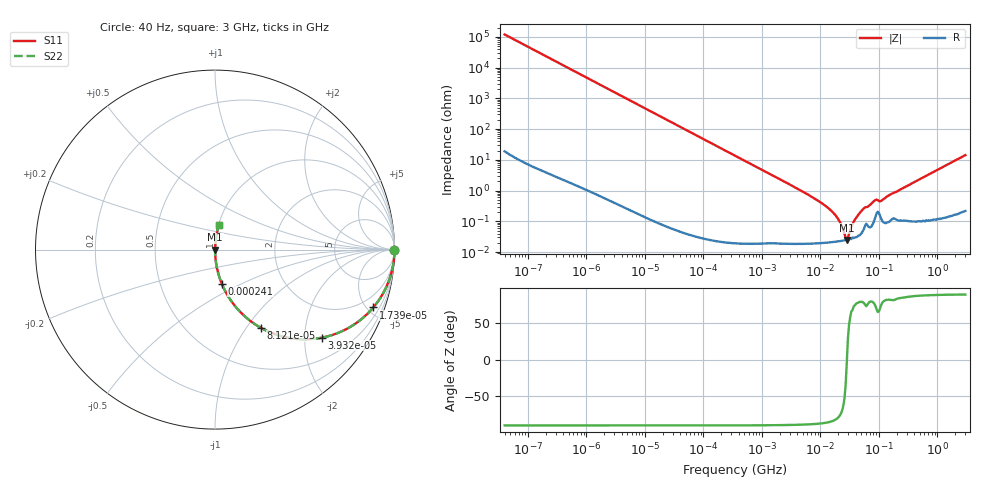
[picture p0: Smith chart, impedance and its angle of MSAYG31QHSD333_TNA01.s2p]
! MSAYG31QHSD333_TNA01  S-PARAMETER MODEL  ( General Type )
! Model Generated by TAIYO YUDEN Corporation (http://www.ty-top.com)
! Version 2.0
! TAIYO YUDEN Control No. 031016
! Copyright(c) 2003 TAIYO YUDEN CO.,LTD. All Rights Reserved.
! Product Description (link to TY-COMPAS)
! https://ds.yuden.co.jp/TYCOMPAS/or/detail?pn=MSAYG31QHSD333KTNA01&u=M
! Products Name : Multilayer Ceramic Capacitors
! Characteristics :
!  Capacitance : 0.033 uF , Rated Voltage : 35V
!  Case Size : 3.2 x 1.6 / 0.126 x 0.063 [mm/inch] , Thickness : 1.15 / 0.045 [mm/inch]
!  (Conditions: Temperature = 25 degC , DC Bias Current/Voltage = 0A / 0V)
! External Node Assignments :
!  1  o---| |---o  2
! GND o---------o GND
! Frequency Range : 40Hz  -  3GHz  [ 401 STEP ]
# MHz S RI R 50
! Freq[MHz].  S11 Real  S11 Imag  S21 Real  S21 Imag  S12 Real  S12 Imag  S22 Real  S22 Imag
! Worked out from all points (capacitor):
!   401 points, 40 Hz to 3 GHz, reference 50 ohm
!   read as one part in series: C = 33.4 nF near 44 Hz
!   lowest |Z| = 25 mohm at 28.14 MHz (marker M1)
!   series resonance near 28.34 MHz, so ESL is about 940 pH
!   S11 on the Smith chart (normalised r, x): 40 Hz: open; 17.39 kHz: 1.00, -5.48; 39.32 kHz: 1.00, -2.42; 81.21 kHz: 1.00, -1.17; 241 kHz: 1.00, -0.39; 3 GHz: 1.00, +0.28
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4e-05  1 -0.00084  8.39e-07 0.00084  8.39e-07 0.00084  1 -0.00084
0.000834  0.9997 -0.0175  0.000311 0.0175  0.000311 0.0175  0.9997 -0.0175
0.004886  0.9895 -0.1016  0.0105 0.1016  0.0105 0.1016  0.9895 -0.1016
0.017386  0.8822 -0.3222  0.1178 0.3222  0.1178 0.3222  0.8822 -0.3222
0.039317  0.5944 -0.4908  0.4056 0.4908  0.4056 0.4908  0.5944 -0.4908
0.081206  0.2558 -0.4361  0.7442 0.4361  0.7442 0.4361  0.2558 -0.4361
0.133706  0.1126 -0.3158  0.8874 0.3158  0.8874 0.3158  0.1126 -0.3158
0.24104  0.0377 -0.19  0.9623 0.19  0.9623 0.19  0.0377 -0.19
0.362475  0.0171 -0.129  0.9829 0.129  0.9829 0.129  0.0171 -0.129
7.222098  0.000226 -0.00615  0.9998 0.00615  0.9998 0.00615  0.000226 -0.00615
11.89125  0.000211 -0.00329  0.9998 0.00329  0.9998 0.00329  0.000211 -0.00329
17.08948  0.000217 -0.00177  0.9998 0.00177  0.9998 0.00177  0.000217 -0.00177
21.43715  0.000228 -0.000934  0.9998 0.000934  0.9998 0.000934  0.000228 -0.000934
25.69909  0.000241 -0.000325  0.9998 0.000325  0.9998 0.000325  0.000241 -0.000325
28.13798  0.000249 -2.52e-05  0.9998 2.52e-05  0.9998 2.52e-05  0.000249 -2.52e-05
30.80834  0.000258 0.000283  0.9997 -0.000283  0.9997 -0.000283  0.000258 0.000283
38.64618  0.0003 0.00108  0.9997 -0.00108  0.9997 -0.00108  0.0003 0.00108
53.07868  0.00049 0.0024  0.9995 -0.0024  0.9995 -0.0024  0.00049 0.0024
83.52119  0.00111 0.00452  0.9989 -0.00452  0.9989 -0.00452  0.00111 0.00452
109.6283  0.00121 0.00449  0.9988 -0.00449  0.9988 -0.00449  0.00121 0.00449
150.5692  0.00102 0.00704  0.999 -0.00704  0.999 -0.00704  0.00102 0.00704
3000  0.0219 0.1389  0.9781 -0.1389  0.9781 -0.1389  0.0219 0.1389
